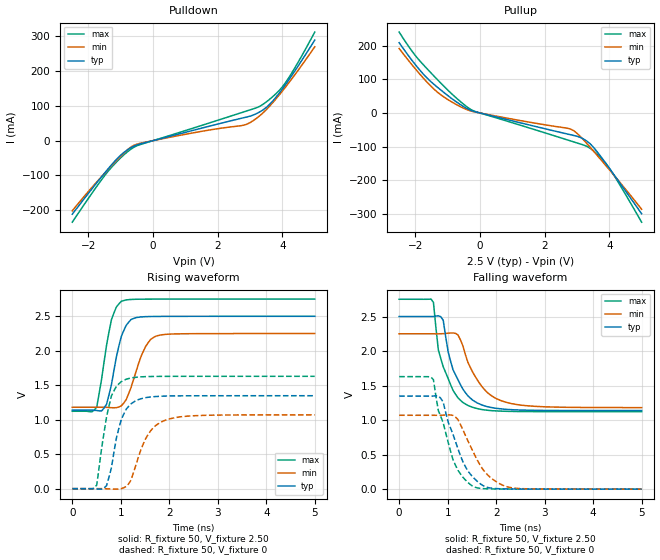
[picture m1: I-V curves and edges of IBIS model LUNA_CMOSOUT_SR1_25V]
[IBIS Ver]   3.2
[Comment Char]   |_char
[File name]   sg8201cga_25v_d.ibs
[File Rev]   1.1
[Date]   2021/10/19 9:35:58
[Source]
[Notes]
[Disclaimer]
This information is for modeling purposes only, and is not guaranteed.
Property of SEIKO EPSON Corp.,
unauthorized reproduction and/or distribution is strictly prohibited.
[Copyright]
Copyright 2021, SEIKO EPSON Corp.
[Component]   2G005_2016
Si_location Pin
Timing_location Pin
[Manufacturer]   SEIKO EPSON Corp.
| 2016 PKG
[Package]
R_pkg   42m   NA   NA
L_pkg   0.49n   NA   NA
C_pkg   0.178p   NA   NA
[Pin] signal_name   model_name
1   OE   NC
2   GND   GND
3   OUT   LUNA_CMOSOUT_SR1_25V
4   VCC   POWER
| Models and submodels in the file (1): LUNA_CMOSOUT_SR1_25V (Output)
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[Model]   LUNA_CMOSOUT_SR1_25V
Model_type Output
Polarity Non-Inverting
Vmeas=1.25
C_comp   2.5p   2.0p   3.0p
[Temperature Range] 25   140   -40
[Voltage Range]   2.50   2.25   2.75
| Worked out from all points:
|   slope of the pulldown table from 0 to 0.375 V, typ, clamps not added: 41.9 ohm
|   slope of the pullup table from 0 to 0.375 V, typ, clamps not added: 42.8 ohm
|   falling waveform, R_fixture 50, V_fixture 2.50: 20-80 % time 397ps typ, 497ps min, 355ps max; typ from 2.5 V to 1.14 V
|   falling waveform, R_fixture 50, V_fixture 0: 20-80 % time 440ps typ, 496ps min, 407ps max; typ from 1.35 V to 0 V
|   rising waveform, R_fixture 50, V_fixture 2.50: 20-80 % time 248ps typ, 323ps min, 230ps max; typ from 1.14 V to 2.5 V
|   rising waveform, R_fixture 50, V_fixture 0: 20-80 % time 265ps typ, 383ps min, 237ps max; typ from 0 V to 1.35 V
[Pullup]
-2.5V     208.9mA    191.8mA    240.5mA
-2V       143.8mA    131.2mA    170.9mA
-1.4V     83.25mA    68.93mA    107.5mA
-900mV    44.71mA    34.39mA    59.2mA
-300mV    8.215mA    6.346mA    11.33mA
2.8V      -64.69mA   -47.74mA   -83.02mA
3V        -69.28mA   -60.33mA   -89.1mA
3.3V      -83.2mA    -90.3mA    -98.96mA
3.6V      -112.5mA   -123.2mA   -119.9mA
3.9V      -150.9mA   -157.1mA   -150.8mA
4.3V      -204.7mA   -203.1mA   -209.6mA
5V        -299.6mA   -286.4mA   -324.7mA
[Pulldown]
-2.5V     -211.8mA   -202mA     -234.7mA
-1.4V     -82.17mA   -83.78mA   -89.22mA
-1V       -41.64mA   -44.57mA   -49.23mA
-600mV    -15.93mA   -13.64mA   -19.31mA
1.2V      28.69mA    21.7mA     34.82mA
2.8V      65.8mA     44.34mA    82.53mA
3.1V      73.65mA    57.69mA    91.49mA
3.4V      88.31mA    79.89mA    104.5mA
3.7V      114mA      109.1mA    126.5mA
4.1V      161.8mA    154.6mA    167.4mA
4.5V      216.8mA    204.2mA    227.8mA
5V        289.2mA    270mA      312.3mA
[Falling Waveform]
R_fixture=50
V_fixture=2.50
V_fixture_min=2.25
V_fixture_max=2.75
0s        2.5V       2.25V      2.75V
707.1ps   2.501V     2.25V      2.704V
808.1ps   2.51V      2.249V     2.019V
909.1ps   2.445V     2.252V     1.771V
1.111ns   1.729V     2.262V     1.431V
1.212ns   1.586V     2.234V     1.324V
1.414ns   1.354V     1.843V     1.214V
1.768ns   1.205V     1.436V     1.147V
2.222ns   1.155V     1.255V     1.127V
5ns       1.139V     1.181V     1.123V
[Falling Waveform]
R_fixture=50
V_fixture=0
V_fixture_min=0
V_fixture_max=0
0s        1.348V     1.07V      1.63V
707.1ps   1.348V     1.07V      1.585V
808.1ps   1.351V     1.07V      1.139V
909.1ps   1.259V     1.072V     958.3mV
1.111ns   792.4mV    1.068V     426.9mV
1.313ns   398.9mV    862.9mV    174.6mV
1.515ns   179.3mV    556.5mV    43.73mV
1.818ns   25.72mV    210.4mV    5.381mV
2.273ns   3.417mV    27.19mV    1.507mV
5ns       437.8uV    743uV      277.7uV
[Rising Waveform]
R_fixture=50
V_fixture=2.50
V_fixture_min=2.25
V_fixture_max=2.75
0s        1.139V     1.181V     1.123V
404ps     1.139V     1.181V     1.114V
505.1ps   1.134V     1.181V     1.186V
707.1ps   1.225V     1.179V     2.082V
808.1ps   1.51V      1.174V     2.452V
1.01ns    2.207V     1.201V     2.717V
1.212ns   2.453V     1.469V     2.745V
1.465ns   2.493V     1.992V     2.748V
1.717ns   2.498V     2.21V      2.749V
5ns       2.5V       2.25V      2.75V
[Rising Waveform]
R_fixture=50
V_fixture=0
V_fixture_min=0
V_fixture_max=0
0s        0V         0V         0V
505.1ps   -3.219mV   266.9uV    52.98mV
707.1ps   44mV       -1.448mV   1.042V
858.6ps   525.8mV    -6.656mV   1.419V
1.01ns    1.002V     1.091mV    1.552V
1.111ns   1.151V     31.18mV    1.587V
1.212ns   1.231V     125.5mV    1.606V
1.515ns   1.321V     728.6mV    1.625V
1.919ns   1.343V     993.4mV    1.629V
5ns       1.348V     1.07V      1.63V
[Ramp]
R_load=50
dV/dt_r   8.088E-1/2.601E-10   6.422E-1/3.833E-10   9.778E-1/2.339E-10
dV/dt_f   8.168E-1/3.974E-10   6.412E-1/4.969E-10   9.764E-1/3.512E-10
|[End   LUNA_CMOSOUT_SR1_25V
